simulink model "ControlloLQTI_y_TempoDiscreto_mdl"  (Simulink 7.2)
settings: Solver=ode45  StartTime=0.0  StopTime=10.0  RelTol=1e-3
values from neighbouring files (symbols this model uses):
  G = chol(Q)    [RegolazioneOttimaTempoInfinita_Integrale.m]    (also in RegolazioneOttimaTempoInfinita_uscita.m; RegolazioneOttimaTempoInfinita_uscita_osservatore.m; RegolazioneOttimaTempoInfinita.m)
  Kyud = -inv(H*inv(F-G*Kd-eye(2))*G)    [ControlloOttimoTempoInfinito_TempoDiscreto.m]
  Ts = 0.01    [RegolazioneOttimaTempoInfinita_TempoDiscreto.m]    (also in ControlloOttimoTempoInfinito_TempoDiscreto.m)
  X0 = [2;-3]    [RegolazioneOttimaTempoInfinita_Integrale.m]    (also in RegolazioneOttimaTempoInfinita_TempoDiscreto.m; RegolazioneOttimaTempoInfinita_uscita.m; RegolazioneOttimaTempoInfinita_uscita_osservatore.m; RegolazioneOttimaTempoInfinita.m)
  yp = 4    [ControlloOttimoTempoInfinito.m]    (also in ControlloOttimoTempoInfinito_TempoDiscreto.m)
undefined symbols (not defined in the file or in its folder): F, H, Kd

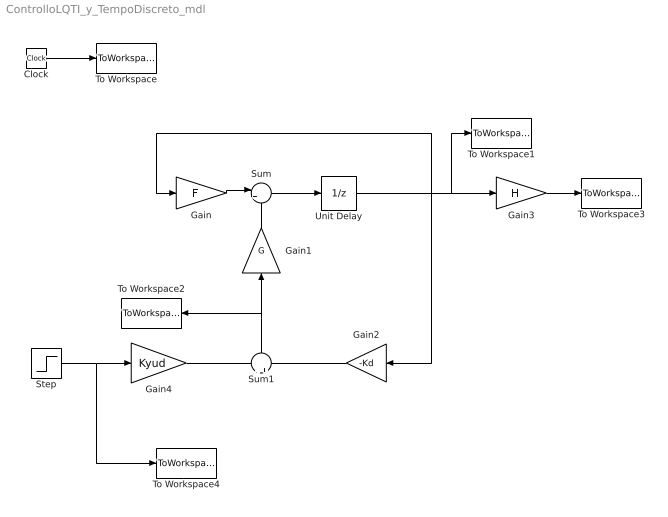
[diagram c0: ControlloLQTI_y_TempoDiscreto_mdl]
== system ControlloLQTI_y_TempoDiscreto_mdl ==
  Clock : Clock
  Gain : Gain  Gain=F  Multiplication=Matrix(K*u)  ParameterDataType=sfix(16)  ParameterScaling=2^0  OutDataType=sfix(16)  OutScaling=2^0
  Gain1 : Gain  Orientation=up  Gain=G  Multiplication=Matrix(K*u)  ParameterDataType=sfix(16)  ParameterScaling=2^0  OutDataType=sfix(16)  OutScaling=2^0
  Gain2 : Gain  Orientation=left  Gain=-Kd  Multiplication=Matrix(K*u)  ParameterDataType=sfix(16)  ParameterScaling=2^0  OutDataType=sfix(16)  OutScaling=2^0
  Gain3 : Gain  Gain=H  Multiplication=Matrix(K*u)  ParameterDataType=sfix(16)  ParameterScaling=2^0  OutDataType=sfix(16)  OutScaling=2^0
  Gain4 : Gain  Gain=Kyud  Multiplication=Matrix(K*u)  ParameterDataType=sfix(16)  ParameterScaling=2^0  OutDataType=sfix(16)  OutScaling=2^0
  Step : Step  Time=5  After=yp  SampleTime=0
  Sum : Sum  Inputs=|++  OutDataType=sfix(16)  OutScaling=2^0
  Sum1 : Sum  Orientation=up  OutDataType=sfix(16)  OutScaling=2^0
  To Workspace : ToWorkspace  VariableName=time  SampleTime=-1  SaveFormat=Array
  To Workspace1 : ToWorkspace  VariableName=X  SampleTime=-1  SaveFormat=Array
  To Workspace2 : ToWorkspace  VariableName=u  SampleTime=-1  SaveFormat=Array
  To Workspace3 : ToWorkspace  VariableName=y  SampleTime=-1  SaveFormat=Array
  To Workspace4 : ToWorkspace  VariableName=yd  SampleTime=-1  SaveFormat=Array
  Unit Delay : UnitDelay  X0=X0  SampleTime=Ts
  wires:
  Gain/1 -> Sum/1
  Unit Delay/1 -> Gain/1, Gain2/1, To Workspace1/1, Gain3/1
  Gain1/1 -> Sum/2
  Sum/1 -> Unit Delay/1
  Clock/1 -> To Workspace/1
  Gain3/1 -> To Workspace3/1
  Sum1/1 -> Gain1/1, To Workspace2/1
  Gain2/1 -> Sum1/2
  Gain4/1 -> Sum1/1
  Step/1 -> Gain4/1, To Workspace4/1
